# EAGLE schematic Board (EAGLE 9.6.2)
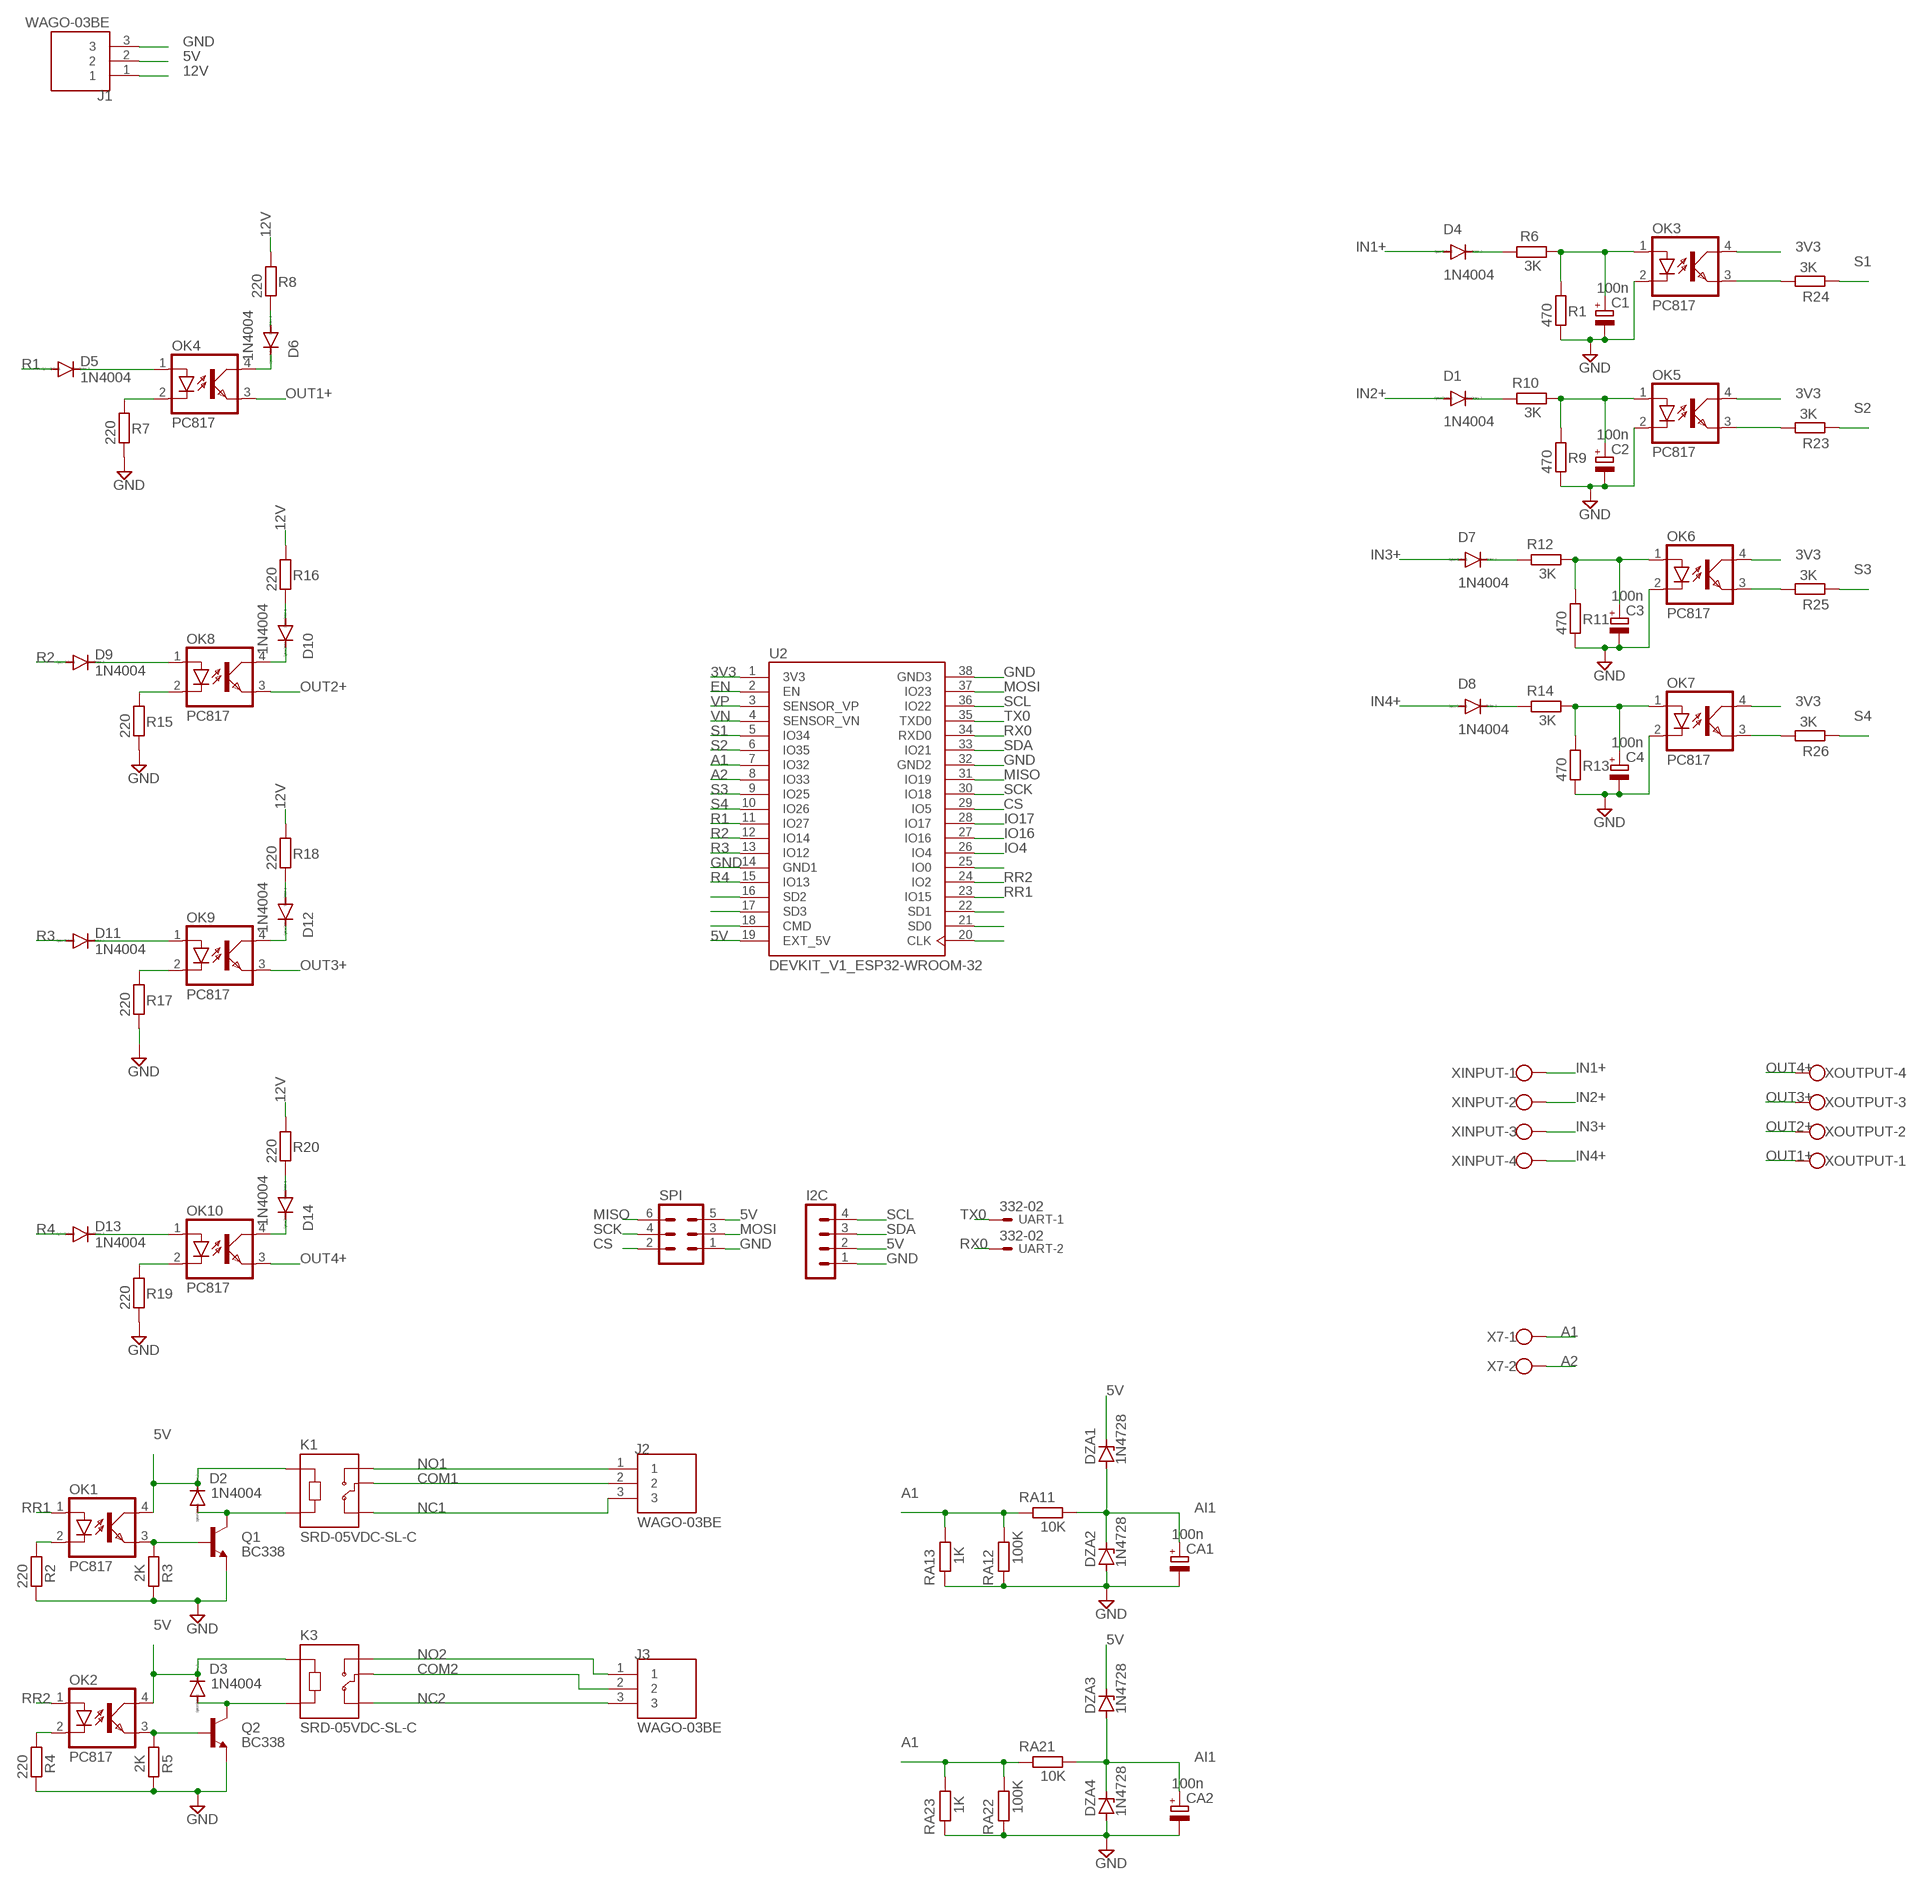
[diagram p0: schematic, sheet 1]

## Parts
C1  100n  CPOL-EUE3.5-8  [E3,5-8]
C2  100n  CPOL-EUE3.5-8  [E3,5-8]
C3  100n  CPOL-EUE3.5-8  [E3,5-8]
C4  100n  CPOL-EUE3.5-8  [E3,5-8]
CA1  100n  CPOL-EUE3.5-8  [E3,5-8]
CA2  100n  CPOL-EUE3.5-8  [E3,5-8]
D1  1N4004  [DO41-10]
D2  1N4004  [DO41-10]
D3  1N4004  [DO41-10]
D4  1N4004  [DO41-10]
D5  1N4004  [DO41-10]
D6  1N4004  [DO41-10]
D7  1N4004  [DO41-10]
D8  1N4004  [DO41-10]
D9  1N4004  [DO41-10]
D10  1N4004  [DO41-10]
D11  1N4004  [DO41-10]
D12  1N4004  [DO41-10]
D13  1N4004  [DO41-10]
D14  1N4004  [DO41-10]
DZA1  1N4728  [DO41Z10]
DZA2  1N4728  [DO41Z10]
DZA3  1N4728  [DO41Z10]
DZA4  1N4728  [DO41Z10]
I2C  MA04-1  [MA04-1]
J1  WAGO-03BE  [CUI_TB006-508-03BE]
J2  WAGO-03BE  [CUI_TB006-508-03BE]
J3  WAGO-03BE  [CUI_TB006-508-03BE]
K1  SRD-05VDC-SL-C  [RELAY_SRD-05VDC-SL-C]
K3  SRD-05VDC-SL-C  [RELAY_SRD-05VDC-SL-C]
OK1  PC817  [DIL04]
OK2  PC817  [DIL04]
OK3  PC817  [DIL04]
OK4  PC817  [DIL04]
OK5  PC817  [DIL04]
OK6  PC817  [DIL04]
OK7  PC817  [DIL04]
OK8  PC817  [DIL04]
OK9  PC817  [DIL04]
OK10  PC817  [DIL04]
Q1  BC338  [TO92-EBC]
Q2  BC338  [TO92-EBC]
R1  470  R-EU_0207/10  [0207/10]
R2  220  R-EU_0207/10  [0207/10]
R3  2K  R-EU_0207/10  [0207/10]
R4  220  R-EU_0207/10  [0207/10]
R5  2K  R-EU_0207/10  [0207/10]
R6  3K  R-EU_0207/10  [0207/10]
R7  220  R-EU_0207/10  [0207/10]
R8  220  R-EU_0207/10  [0207/10]
R9  470  R-EU_0207/10  [0207/10]
R10  3K  R-EU_0207/10  [0207/10]
R11  470  R-EU_0207/10  [0207/10]
R12  3K  R-EU_0207/10  [0207/10]
R13  470  R-EU_0207/10  [0207/10]
R14  3K  R-EU_0207/10  [0207/10]
R15  220  R-EU_0207/10  [0207/10]
R16  220  R-EU_0207/10  [0207/10]
R17  220  R-EU_0207/10  [0207/10]
R18  220  R-EU_0207/10  [0207/10]
R19  220  R-EU_0207/10  [0207/10]
R20  220  R-EU_0207/10  [0207/10]
R23  3K  R-EU_0207/10  [0207/10]
R24  3K  R-EU_0207/10  [0207/10]
R25  3K  R-EU_0207/10  [0207/10]
R26  3K  R-EU_0207/10  [0207/10]
RA11  10K  R-EU_0207/10  [0207/10]
RA12  100K  R-EU_0207/10  [0207/10]
RA13  1K  R-EU_0207/10  [0207/10]
RA21  10K  R-EU_0207/10  [0207/10]
RA22  100K  R-EU_0207/10  [0207/10]
RA23  1K  R-EU_0207/10  [0207/10]
SPI  MA03-2  [MA03-2]
U2  DEVKIT_V1_ESP32-WROOM-32  [MODULE_DEVKIT_V1_ESP32-WROOM-32]
UART  332-02  [332-02]
X7  W237-102  [W237-102]
XINPUT  W237-4  [W237-4]
XOUTPUT  W237-4  [W237-4]

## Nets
3V3: OK3.4(COL) OK5.4(COL) OK6.4(COL) OK7.4(COL) U2.1(3V3)
5V: D2.C D3.C DZA1.C DZA3.C I2C.2 J1.2 K1.A1 K3.A1 OK1.4(COL) OK2.4(COL) SPI.5 U2.19(EXT_5V)
12V: J1.1 R8.1 R16.1 R18.1 R20.1
A1: RA11.1 RA12.2 RA13.2 RA21.1 RA22.2 RA23.2 U2.7(IO32) X7.1
A2: U2.8(IO33) X7.2
AI1: CA1.+ CA2.+ DZA1.A DZA2.C DZA3.A DZA4.C RA11.2 RA21.2
COM1: J2.2 K1.COM
COM2: J3.2 K3.COM
CS: SPI.2 U2.29(IO5)
EN: U2.2(EN)
GND: C1.- C2.- C3.- C4.- CA1.- CA2.- DZA2.A DZA4.A I2C.1 J1.3 OK3.2(C) OK5.2(C) OK6.2(C) OK7.2(C) Q1.E Q2.E R1.2 R2.2 R3.2 R4.2 R5.2 R7.2 R9.2 R11.2 R13.2 R15.2 R17.2 R19.2 RA12.1 RA13.1 RA22.1 RA23.1 SPI.1 U2.14(GND1) U2.32(GND2) U2.38(GND3)
IN1+: D4.A XINPUT.1
IN2+: D1.A XINPUT.2
IN3+: D7.A XINPUT.3
IN4+: D8.A XINPUT.4
IO4: U2.26(IO4)
IO16: U2.27(IO16)
IO17: U2.28(IO17)
MISO: SPI.6 U2.31(IO19)
MOSI: SPI.3 U2.37(IO23)
N$1: OK2.2(C) R4.1
N$2: OK1.2(C) R2.1
N$3: OK1.3(EMIT) Q1.B R3.1
N$4: D2.A K1.A2 Q1.C
N$5: OK5.3(EMIT) R23.2
N$6: OK2.3(EMIT) Q2.B R5.1
N$7: D3.A K3.A2 Q2.C
N$8: OK3.3(EMIT) R24.2
N$9: C1.+ OK3.1(A) R1.1 R6.2
N$10: D5.C OK4.1(A)
N$11: D4.C R6.1
N$12: OK4.2(C) R7.1
N$13: D6.A R8.2
N$14: C2.+ OK5.1(A) R9.1 R10.2
N$15: D1.C R10.1
N$16: C3.+ OK6.1(A) R11.1 R12.2
N$17: D7.C R12.1
N$18: C4.+ OK7.1(A) R13.1 R14.2
N$19: D8.C R14.1
N$20: D9.C OK8.1(A)
N$21: OK8.2(C) R15.1
N$22: D10.A R16.2
N$23: D11.C OK9.1(A)
N$24: OK9.2(C) R17.1
N$25: D12.A R18.2
N$26: D13.C OK10.1(A)
N$27: OK10.2(C) R19.1
N$28: D14.A R20.2
N$29: D12.C OK9.4(COL)
N$44: U2.16(SD2)
N$45: U2.17(SD3)
N$46: U2.18(CMD)
N$49: OK6.3(EMIT) R25.2
N$50: OK7.3(EMIT) R26.2
N$52: D14.C OK10.4(COL)
N$53: D10.C OK8.4(COL)
N$55: D6.C OK4.4(COL)
N$61: U2.25(IO0)
N$64: U2.22(SD1)
N$65: U2.21(SD0)
N$66: U2.20(CLK)
NC1: J2.3 K1.NC
NC2: J3.3 K3.NC
NO1: J2.1 K1.NO
NO2: J3.1 K3.NO
OUT1+: OK4.3(EMIT) XOUTPUT.1
OUT2+: OK8.3(EMIT) XOUTPUT.2
OUT3+: OK9.3(EMIT) XOUTPUT.3
OUT4+: OK10.3(EMIT) XOUTPUT.4
R1: D5.A U2.11(IO27)
R2: D9.A U2.12(IO14)
R3: D11.A U2.13(IO12)
R4: D13.A U2.15(IO13)
RR1: OK1.1(A) U2.23(IO15)
RR2: OK2.1(A) U2.24(IO2)
RX0: U2.34(RXD0) UART.2
S1: R24.1 U2.5(IO34)
S2: R23.1 U2.6(IO35)
S3: R25.1 U2.9(IO25)
S4: R26.1 U2.10(IO26)
SCK: SPI.4 U2.30(IO18)
SCL: I2C.4 U2.36(IO22)
SDA: I2C.3 U2.33(IO21)
TX0: U2.35(TXD0) UART.1
VN: U2.4(SENSOR_VN)
VP: U2.3(SENSOR_VP)

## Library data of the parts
C1-C4 CA1 CA2 = rcl:CPOL-EU: POLARIZED CAPACITOR, European symbol; SPICEPREFIX: C
D1-D14 = diode:1N4004: DIODE
DZA1-DZA4 = diode:1N4728: Z DIODE
I2C = con-lstb:MA04-1: PIN HEADER; OC_FARNELL: unknown; OC_NEWARK: unknown
J1-J3 = TB006-508-03BE:WAGO-03BE: Check availability; AVAILABILITY: In Stock; CHECK_PRICES: https://www.snapeda.com/parts/TB006-508-03BE/Same+Sky/view-part/?ref=eda; DESCRIPTION: 2~24 Poles, Screw Type, Horizontal, 5.08 Pitch, 26~14 (AWG), Terminal Block Connector; MF: Same Sky; MP: TB006-508-03BE; PACKAGE: None; PRICE: None; SNAPEDA_LINK: https://www.snapeda.com/parts/TB006-508-03BE/Same+Sky/view-part/?ref=snap
K1 K3 = SRD-05VDC-SL-C:SRD-05VDC-SL-C: 5V Trigger Relay Module For Arduino And Raspberry Pi 5V Trigger Relay Module For Arduino And Raspberry Pi Check availability; AVAILABILITY: In Stock; CHECK_PRICES: https://www.snapeda.com/parts/SRD-05VDC-SL-C/Songle+Relay/view-part/?ref=eda; DESCRIPTION: 5V Trigger Relay Module For Arduino And Raspberry Pi 5V Trigger Relay Module For Arduino And Raspberry Pi; MF: Songle Relay; MP: SRD-05VDC-SL-C; PACKAGE: NON STANDARD-5 Songle Relay; PRICE: None; SNAPEDA_LINK: https://www.snapeda.com/parts/SRD-05VDC-SL-C/Songle+Relay/view-part/?ref=snap
OK1-OK10 = optocoupler:PC817: SHARP OPTO COUPLER; MPN: PC817X4J000F; OC_FARNELL: 9707727; OC_NEWARK: 97K7059
Q1 Q2 = transistor-npn:BC338*: NPN Transistor
R1-R20 R23-R26 RA11-RA13 RA21-RA23 = rcl:R-EU_: RESISTOR, European symbol; SPICEPREFIX: R
SPI = con-lstb:MA03-2: PIN HEADER; OC_FARNELL: unknown; OC_NEWARK: unknown
U2 = DEVKIT_V1_ESP32-WROOM-32:DEVKIT_V1_ESP32-WROOM-32: Check availability; AVAILABILITY: Not in stock; CHECK_PRICES: https://www.snapeda.com/parts/DEVKIT%20V1%20ESP32-WROOM-32/Espressif+Systems/view-part/?ref=eda; DESCRIPTION: WROOM-32 Development Board ESP32 ESP-32S WiFi Bluetooth Dev Module; MF: Espressif Systems; MP: DEVKIT V1 ESP32-WROOM-32; PACKAGE: Package; PRICE: None; SNAPEDA_LINK: https://www.snapeda.com/parts/DEVKIT%20V1%20ESP32-WROOM-32/Espressif+Systems/view-part/?ref=snap
UART = con-garry:332-02: 2 Pin - 2mm Dual Row
X7 = con-wago-500:W237-102: WAGO SCREW CLAMP; MPN: 237-102; OC_FARNELL: unknown; OC_NEWARK: 70K9898
XINPUT XOUTPUT = con-wago-500:W237-4: WAGO SCREW CLAMP; OC_FARNELL: unknown; OC_NEWARK: unknown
